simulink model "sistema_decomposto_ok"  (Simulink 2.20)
settings: Solver=ode45  StartTime=0.0  StopTime=10.0  RelTol=1e-3  AbsTol=1e-6

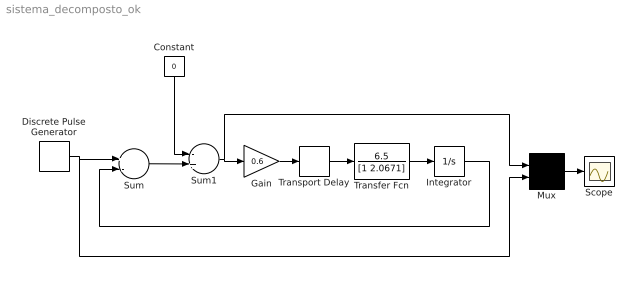
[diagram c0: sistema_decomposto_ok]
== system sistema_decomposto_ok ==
  Constant : Constant  Orientation=down  Value=0
  Discrete Pulse Generator : DiscretePulseGenerator  Amplitude=47.5  Period=100  PulseWidth=100  PhaseDelay=10  SampleTime=.1
  Gain : Gain  Gain=0.6
  Integrator : Integrator  ExternalReset=none  InitialConditionSource=internal  InitialCondition=0  LimitOutput=off  UpperSaturationLimit=inf  LowerSaturationLimit=-inf  ShowSaturationPort=off  ShowStatePort=off  AbsoluteTolerance=auto
  Mux : Mux  Inputs=2
  Scope : Scope
  Sum : Sum  Inputs=+-
  Sum1 : Sum  Inputs=-+
  Transfer Fcn : TransferFcn  Numerator=6.5  Denominator=[1 2.0671]
  Transport Delay : TransportDelay  DelayTime=.190  InitialInput=0  BufferSize=1024
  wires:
  Mux/1 -> Scope/1
  Discrete Pulse Generator/1 -> Sum/1, Mux/2
  Transfer Fcn/1 -> Integrator/1
  Transport Delay/1 -> Transfer Fcn/1
  Sum/1 -> Sum1/2
  Constant/1 -> Sum1/1
  Gain/1 -> Transport Delay/1
  Integrator/1 -> Sum/2
  Sum1/1 -> Gain/1, Mux/1
